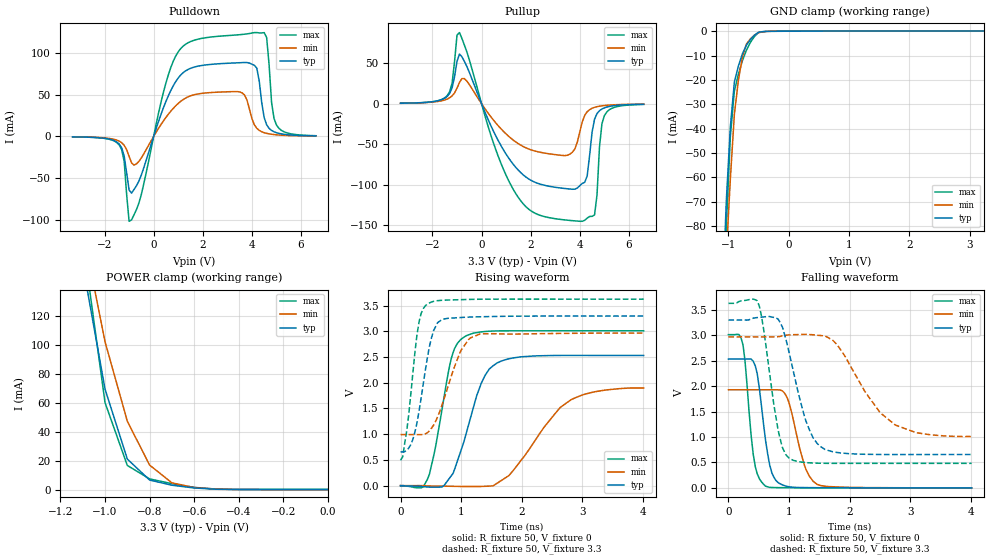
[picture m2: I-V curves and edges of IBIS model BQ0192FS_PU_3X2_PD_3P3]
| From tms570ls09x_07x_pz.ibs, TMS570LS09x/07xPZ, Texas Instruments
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|   Model Cell BQ0192FS_PU_3X2_PD_3P3
|BQ0192FS_PU_3X2_PD_3P3
[Model]   BQ0192FS_PU_3X2_PD_3P3
Model_type   I/O
Polarity   Non-Inverting
Enable   Active-Low
Vinl =  1.25
Vinh =  1.65
Cref =  15.0001pF
Rref =  101.0000M
Vref =  0V
Vmeas =  1.65
C_comp   1.2p   1.2p   1.2p
[Model Spec]
Vinl   1.25   1.12   1.38
Vinh   1.65   1.45   1.75
[Temperature Range]   25   155   -40
[Voltage Range]   3.3   2.97   3.63
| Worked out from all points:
|   slope of the pulldown table from 0 to 0.495 V, typ, clamps not added: 11.9 ohm
|   slope of the pullup table from 0 to 0.495 V, typ, clamps not added: 14.3 ohm
|   GND clamp passes 1 mA (typ) near -0.53 V on its own axis
|   POWER clamp passes 1 mA (typ) near -0.58 V on its own axis
|   rising waveform, R_fixture 50, V_fixture 0: 20-80 % time 400ps typ, 718ps min, 275ps max; typ from 0 V to 2.53 V
|   rising waveform, R_fixture 50, V_fixture 3.3: 20-80 % time 225ps typ, 347ps min, 172ps max; typ from 0.656 V to 3.3 V
|   falling waveform, R_fixture 50, V_fixture 0: 20-80 % time 170ps typ, 243ps min, 138ps max; typ from 2.53 V to 0 V
|   falling waveform, R_fixture 50, V_fixture 3.3: 20-80 % time 342ps typ, 655ps min, 230ps max; typ from 3.3 V to 0.656 V
[POWER_clamp]
|   voltage   I(typ)   I(min)   I(max)
-3.3V     2.375A     2.63A      3.153A
-1.1V     156mA      180.2mA    173.4mA
-1.067V   127.2mA    154.3mA    135.7mA
-1.033V   98.46mA    128.4mA    98.04mA
-1V       69.67mA    102.5mA    60.33mA
-900mV    21.21mA    47.43mA    16.77mA
-800mV    6.67mA     17.03mA    7.475mA
-700mV    3.094mA    4.728mA    4.157mA
-600mV    1.183mA    1.448mA    1.593mA
-500mV    283.5uA    402.1uA    371.9uA
0V        96.5uA     44.21uA    168.6uA
[Pulldown]
|   voltage   I(typ)   I(min)   I(max)
-3.3V     -554.3uA   -511.5uA   -526.2uA
-1.4V     -9.291mA   -5.703mA   -10.34mA
-1.2V     -23.68mA   -10.64mA   -30.19mA
-1V       -64.35mA   -24mA      -101.9mA
-600mV    -53.61mA   -29.92mA   -79.97mA
1V        70.15mA    39.6mA     101.5mA
3.5V      88.44mA    53.42mA    122.1mA
4.2V      81.93mA    9.711mA    124.7mA
4.6V      13.96mA    3.646mA    118.8mA
4.8V      7.183mA    2.57mA     41.14mA
5V        4.453mA    1.905mA    13.75mA
6.6V      621.1uA    479.2uA    840.9uA
[Pullup]
|   voltage   I(typ)   I(min)   I(max)
-3.3V     614.6uA    591.9uA    551.1uA
-1.4V     9.028mA    5.738mA    10.01mA
-900mV    61.33mA    26.24mA    87.8mA
1.4V      -78.76mA   -47.33mA   -111.2mA
3.5V      -105mA     -63.56mA   -143.7mA
4.1V      -98.29mA   -22.39mA   -145.1mA
4.3V      -89.13mA   -9.839mA   -141.1mA
4.6V      -19.02mA   -4.469mA   -137.2mA
4.7V      -12.15mA   -3.653mA   -112.5mA
4.8V      -8.616mA   -3.042mA   -53.65mA
5V        -5.089mA   -2.205mA   -14.76mA
6.6V      -663.5uA   -536.5uA   -825.6uA
[GND_clamp]
|   voltage   I(typ)   I(min)   I(max)
-3.3V     -1.947A    -1.623A    -3.254A
-1.1V     -112mA     -127.1mA   -135.8mA
-1.033V   -69.62mA   -91.64mA   -80.2mA
-966.7mV  -39.25mA   -60.63mA   -43.13mA
-900mV    -20.89mA   -34.03mA   -24.55mA
-833.3mV  -14.3mA    -20.13mA   -17.67mA
-766.7mV  -9.242mA   -10.53mA   -12.09mA
-700mV    -5.726mA   -5.229mA   -7.796mA
-566.7mV  -1.616mA   -1.599mA   -2.13mA
-500mV    -447.1uA   -610.1uA   -527.1uA
-300mV    -27.38uA   -21.6uA    -40.6uA
3.233V    96.49uA    48.22uA    168.5uA
[Ramp]
| variable   typ   min   max
dV/dt_f   1.63014/0.3484835n   1.216799/0.6765226n   1.938925/0.2336543n
dV/dt_r   1.539219/0.401855n   1.169604/0.7486661n   1.834583/0.2784518n
R_load = 50
[Rising Waveform]
R_fixture = 50
V_fixture = 0
V_fixture_min = 0
V_fixture_max = 0
|   time   V(typ)   V(min)   V(max)
0s        299.8uV    -942.5nV   -9.813mV
340ps     -15.6mV    -293.9uV   -44.72mV
444ps     -27.28mV   -6.965mV   122mV
580ps     -31.67mV   -9.747mV   766.4mV
840ps     194.5mV    -13.93mV   2.484V
1.072ns   964.8mV    -18.17mV   2.908V
1.332ns   1.99V      -17.6mV    2.991V
1.656ns   2.42V      92.99mV    3.011V
2.808ns   2.533V     1.666V     3.013V
4.012ns   2.532V     1.899V     3.013V
[Rising Waveform]
R_fixture = 50
V_fixture = 3.3
V_fixture_min = 2.97
V_fixture_max = 3.63
|   time   V(typ)   V(min)   V(max)
0s        655.7mV    992.7mV    492.2mV
36ps      654.6mV    992.7mV    561.4mV
104ps     687.3mV    992.7mV    1.077V
204ps     899.8mV    992.8mV    2.197V
308ps     1.467V     991.3mV    3.198V
444ps     2.494V     1.029V     3.535V
612ps     3.171V     1.339V     3.599V
972ps     3.269V     2.562V     3.617V
1.152ns   3.28V      2.874V     3.624V
4.012ns   3.299V     2.968V     3.629V
[Falling Waveform]
R_fixture = 50
V_fixture = 0
V_fixture_min = 0
V_fixture_max = 0
|   time   V(typ)   V(min)   V(max)
0s        2.532V     1.929V     3.013V
240ps     2.532V     1.929V     2.815V
408ps     2.492V     1.929V     668.2mV
476ps     2.237V     1.929V     272.9mV
612ps     938.2mV    1.929V     33.45mV
716ps     296.7mV    1.929V     7.313mV
944ps     36.23mV    1.827V     3.344mV
1.256ns   5.51mV     437.1mV    1.065mV
1.464ns   3.156mV    67.23mV    659.3uV
4.012ns   96.17uV    776uV      -7.95uV
[Falling Waveform]
R_fixture = 50
V_fixture = 3.3
V_fixture_min = 2.97
V_fixture_max = 3.63
|   time   V(typ)   V(min)   V(max)
0s        3.299V     2.969V     3.629V
476ps     3.348V     2.969V     3.679V
580ps     3.361V     2.969V     3.125V
816ps     3.323V     2.971V     1.161V
892ps     3.158V     2.99V      790.6mV
1.024ns   2.539V     3.01V      566.7mV
1.28ns    1.311V     3.019V     496.5mV
1.592ns   756mV      2.987V     482.9mV
2.752ns   655.3mV    1.237V     482mV
4.012ns   656mV      1.009V     481.7mV
